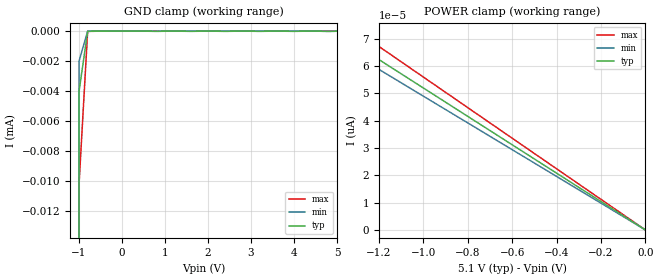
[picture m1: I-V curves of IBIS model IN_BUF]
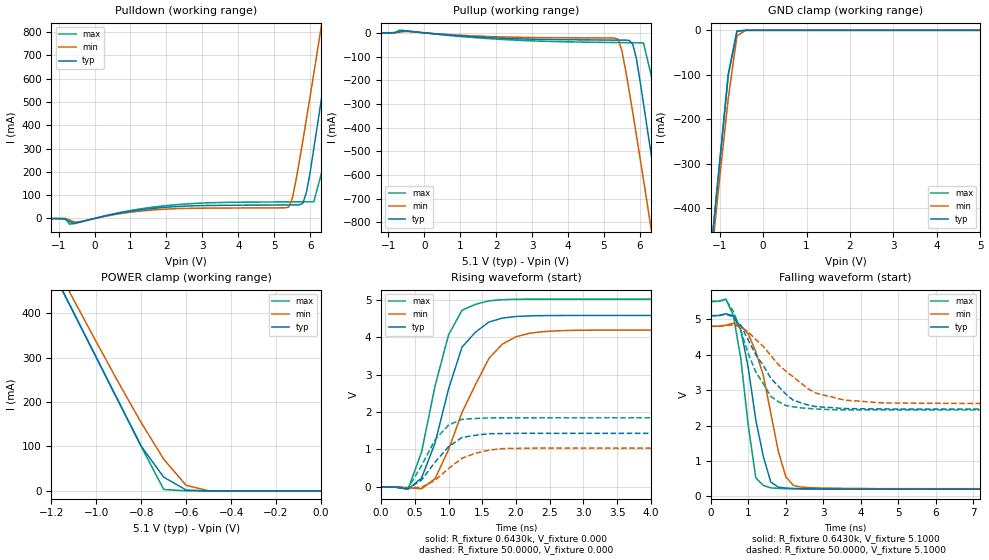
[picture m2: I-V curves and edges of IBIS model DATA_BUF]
| IBIS file m48z02.ibs created by s2ibis2 version 1.1
| North Carolina State University Electronics Research Laboratory  1995
[IBIS ver]   2.1
[File name]   m48z02.ibs
[File Rev]   0
[Date]   May 17, 2002
[Source]   ST models
[Copyright]   ST Microelectronics Inc.
|   Component m48z02 [Package]
[Component]   m48z02 [Package]
[Manufacturer]   ST Microelectronics
[Package]
| variable   typ   min   max
R_pkg   10.0000m   10.0000m   10.0000m
L_pkg   13.0000nH   8.0000nH   18.0000nH
C_pkg   6.0000pF   4.0000pF   8.0000pF
[Pin]  signal_name   model_name   R_pin   L_pin   C_pin
| fdatadummy   dummy
| goe  dummy   dummy
1   A7   IN_BUF
2   A6   IN_BUF
3   A5   IN_BUF
4   A4   IN_BUF
5   A3   IN_BUF
6   A2   IN_BUF
7   A1   IN_BUF
8   A0   IN_BUF
9   DQ0   DATA_BUF
10   DQ1   DATA_BUF
11   DQ2   DATA_BUF
12   VSS   GND
13   DQ3   DATA_BUF
14   DQ4   DATA_BUF
15   DQ5   DATA_BUF
16   DQ6   DATA_BUF
17   DQ7   DATA_BUF
18   E#   IN_BUF
19   A10   IN_BUF
20   G#   IN_BUF
21   W#   IN_BUF
22   A9   IN_BUF
23   A8   IN_BUF
24   VCC   POWER
[Package Model]  PCDIP24
| Models and submodels in the file (2): IN_BUF (Input), DATA_BUF (3-state)
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|   Model IN_BUF
[Model]   IN_BUF
Model_type   Input
Vinl =   0.8000V
Vinh =   2.0000V
C_comp   6.0800pF   5.9900pF   6.2200pF
[Temperature Range]   27.0000   0.000   70.0000
[Voltage Range]   5.1000V   4.8000V   5.5000V
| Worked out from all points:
|   GND clamp passes 1 mA (typ) near -1.03 V on its own axis
[GND_clamp]
| voltage   I(typ)   I(min)   I(max)
-5V       -3.645A    -3.66A     -3.622A
-1.2V     -6.986mA   -7.174mA   -6.983mA
-1V       -4.01uA    -1.994uA   -10.21uA
-800mV    -1.738nA   -399.5pA   -11.69nA
5V        5pA        5pA        372.3pA
[POWER_clamp]
| voltage   I(typ)   I(min)   I(max)
-5V       260pA      245pA      280pA
-1.5V     77.99pA    73.5pA     84pA
-1.4V     72.79pA    68.6pA     78.4pA
-1.3V     67.59pA    63.7pA     72.8pA
0V        0A         0A         0A
|   Model DATA_BUF
[Model]   DATA_BUF
Model_type   3-state
Polarity   Inverting
Enable   Active-Low
Vinl =   0.8000V
Vinh =   2.0000V
Vmeas =   1.5000V
Cref =1.000e-10F
Rref =   0.6430k
Vref =   1.7800V
C_comp   5.7000pF   5.6800pF   5.7700pF
[Temperature Range]   27.0000   0.000   70.0000
[Voltage Range]   5.1000V   4.8000V   5.5000V
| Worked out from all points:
|   slope of the pulldown table from 0 to 0.765 V, typ, clamps not added: 30.6 ohm
|   slope of the pullup table from 0 to 0.765 V, typ, clamps not added: 75.6 ohm
|   GND clamp passes 1 mA (typ) near -0.50 V on its own axis
|   POWER clamp passes 1 mA (typ) near -0.55 V on its own axis
|   rising waveform, R_fixture 0.6430k, V_fixture 0.000: 20-80 % time 442ps typ, 616ps min, 385ps max; typ from 0 V to 4.58 V
|   rising waveform, R_fixture 50.0000, V_fixture 0.000: 20-80 % time 414ps typ, 475ps min, 376ps max; typ from 0 V to 1.43 V
|   falling waveform, R_fixture 0.6430k, V_fixture 5.1000: 20-80 % time 483ps typ, 581ps min, 389ps max; typ from 5.1 V to 0.205 V
|   falling waveform, R_fixture 50.0000, V_fixture 5.1000: 20-80 % time 988ps typ, 1.31ns min, 750ps max; typ from 5.1 V to 2.46 V
[Pulldown]
| voltage   I(typ)   I(min)   I(max)
-5V       0A         0A         0A
-700mV    -12.55mA   -5.568mA   -24.43mA
2V        48.3mA     40.27mA    55.28mA
5.4V      58.03mA    48.56mA    71.33mA
5.5V      58.1mA     85.36mA    71.42mA
5.8V      66.22mA    338.3mA    71.69mA
5.9V      115.2mA    431.8mA    71.78mA
6.1V      300mA      622.3mA    71.99mA
6.5V      700mA      1.01A      300mA
6.9V      1.1A       1.402A     700mA
7.3V      1.5A       1.8A       1.1A
10.1V     4.3A       4.6A       3.9A
[Pullup]
| voltage   I(typ)   I(min)   I(max)
-5V       0A         0A         0A
-700mV    4.754mA    1.888mA    11mA
5.3V      -30.64mA   -21.82mA   -40.9mA
5.4V      -30.73mA   -28.15mA   -41.05mA
5.5V      -30.81mA   -77.35mA   -41.19mA
5.8V      -47.56mA   -336.6mA   -41.6mA
5.9V      -107.6mA   -430.4mA   -41.77mA
6.1V      -300mA     -621.3mA   -42.92mA
6.5V      -700mA     -1.01A     -300mA
6.9V      -1.1A      -1.402A    -700mA
7.3V      -1.5A      -1.8A      -1.1A
10.1V     -4.3A      -4.6A      -3.9A
[GND_clamp]
| voltage   I(typ)   I(min)   I(max)
-5V       -4.3A      -4.3A      -4.3A
-1.2V     -500mA     -524.6mA   -500mA
-1V       -300mA     -335.1mA   -300mA
-800mV    -100.6mA   -153.4mA   -100mA
-600mV    -2.081mA   -12.47mA   -1.528mA
-400mV    -2.338uA   -4.341uA   -113.9uA
5V        8.471nA    1.019nA    24.33nA
[POWER_clamp]
| voltage   I(typ)   I(min)   I(max)
-5V       4.3A       4.3A       4.3A
-1.2V     500mA      524.5mA    500mA
-1.1V     400mA      429.3mA    400mA
-900mV    200mA      242.6mA    200mA
-800mV    100.5mA    153.4mA    100mA
-700mV    30.92mA    71.4mA     3.297mA
-600mV    1.989mA    12.47mA    173.9uA
-500mV    44.72uA    299.1uA    14.9uA
0V        0A         0A         18.94nA
[Ramp]
| variable   typ   min   max
dV/dt_r   2.7484/0.4296n   2.5139/0.5516n   3.0112/0.3615n
dV/dt_f   2.9370/0.4210n   2.7490/0.5410n   3.1770/0.3578n
R_load = 0.6430k
[Rising Waveform]
R_fixture = 0.6430k
V_fixture = 0.000
V_fixture_min = 0.000
V_fixture_max = 0.000
| time   V(typ)   V(min)   V(max)
0s        3.147nV    3.43nV     12.02nV
400ps     -62.44mV   -27.66mV   -62.99mV
600ps     234mV      -51.61mV   928.1mV
800ps     1.169V     216.6mV    2.694V
1ns       2.613V     990.6mV    4.059V
1.2ns     3.734V     1.987V     4.718V
1.4ns     4.135V     2.732V     4.879V
1.8ns     4.51V      3.816V     5.002V
2.4ns     4.576V     4.148V     5.018V
10ns      4.581V     4.19V      5.019V
[Rising Waveform]
R_fixture = 50.0000
V_fixture = 0.000
V_fixture_min = 0.000
V_fixture_max = 0.000
| time   V(typ)   V(min)   V(max)
0s        2.161nV    2.268nV    8.435nV
200ps     -2.961mV   -206.1uV   -8.046mV
400ps     -46.13mV   -21.39mV   -37.13mV
600ps     179mV      -14.51mV   567.6mV
800ps     659.8mV    175.1mV    1.259V
1ns       1.07V      488.7mV    1.65V
1.2ns     1.32V      764.7mV    1.806V
1.4ns     1.378V     897.2mV    1.826V
1.8ns     1.424V     1.022V     1.844V
10ns      1.429V     1.035V     1.845V
[Falling Waveform]
R_fixture = 0.6430k
V_fixture = 5.1000
V_fixture_min = 4.8000
V_fixture_max = 5.5000
| time   V(typ)   V(min)   V(max)
0s        5.1V       4.8V       5.5V
400ps     5.154V     4.83V      5.569V
600ps     5.098V     4.888V     5.111V
800ps     4.7V       4.826V     3.889V
1.2ns     2.158V     4.083V     526.5mV
1.4ns     1.132V     3.418V     310mV
1.6ns     408.4mV    2.352V     242.2mV
1.8ns     262.8mV    1.284V     227mV
2.2ns     226.7mV    312.5mV    214.4mV
10ns      205mV      218.3mV    205.1mV
[Falling Waveform]
R_fixture = 50.0000
V_fixture = 5.1000
V_fixture_min = 4.8000
V_fixture_max = 5.5000
| time   V(typ)   V(min)   V(max)
0s        5.1V       4.8V       5.5V
400ps     5.139V     4.822V     5.545V
600ps     5.068V     4.84V      5.229V
800ps     4.82V      4.778V     4.672V
1.2ns     3.998V     4.426V     3.51V
1.6ns     3.337V     3.976V     2.824V
2ns       2.892V     3.539V     2.566V
2.8ns     2.536V     2.917V     2.469V
3.6ns     2.479V     2.714V     2.442V
10ns      2.465V     2.625V     2.44V
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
